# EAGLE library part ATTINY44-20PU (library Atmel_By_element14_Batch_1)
8-bit Microcontroller with In-System Programmable Flash
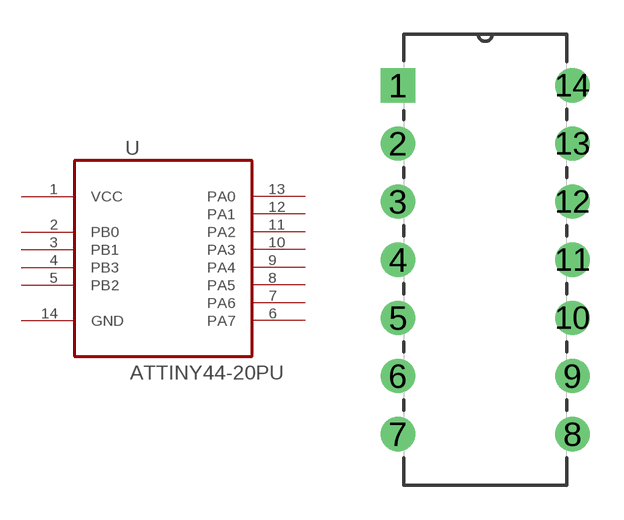
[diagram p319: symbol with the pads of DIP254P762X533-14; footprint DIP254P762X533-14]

Designator prefix U

## ATTINY44-20PU (MPN: ATTINY44-20PU; OC_FARNELL: 1455150; OC_NEWARK: 58M3786; PACKAGE: PDIP-14; SUPPLIER: Atmel)  [DIP254P762X533-14]
1  VCC  pwr
2  PB0
3  PB1
4  PB3
5  PB2
6  PA7
7  PA6
8  PA5
9  PA4
10  PA3
11  PA2
12  PA1
13  PA0
14  GND  pas

## Footprint DIP254P762X533-14 (pad centres in mm)
drill 0.991 square: 1 -7.62,15.24
drill 0.991: 2 -7.62,12.7; 3 -7.62,10.16; 4 -7.62,7.62; 5 -7.62,5.08; 6 -7.62,2.54; 7 -7.62,0; 8 0,0; 9 0,2.54; 10 0,5.08; 11 0,7.62; 12 0,10.16; 13 0,12.7; 14 0,15.24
